FUNCTION_BLOCK "IMAC_STANDBY"
TITLE = STANDBY
//--------------------------------------------------------------------------------
//SIEMENS AG     I&S IP PEP SNPSP-Element: D-09300081-E-E5
//--------------------------------------------------------------------------------
//History
//=======
//  Date    Version  Description                     Author        CheckedReleased
//1997/06/09   0.6   Basic Edition                   Salge
//2004/11/25   1.0   Basic Edition converted to S7   Edelmann
//2004/12/02   1.1   Reset Timer in normal C/O       Edelmann
//--------------------------------------------------------------------------------
//PLC:   >= S7-300
//--------------------------------------------------------------------------------
//Specification:   Refer "TECHFUNK.DOC"
//--------------------------------------------------------------------------------
//Called FC : FC90 "DELAYTIMER"
//            SFC20 "BLKMOV"
//References: DB90.DBX3.1  (1 sec tact)
//--------------------------------------------------------------------------------
//at run time:
//--------------------------------------------------------------------------------
//
//--------------------------------------------------------------------------------
//Note:
//--------------------------------------------------------------------------------
// KNOW_HOW_PROTECT
AUTHOR : Sa_Edm
FAMILY : IMAC
NAME : STANDBY
VERSION : 1.0


VAR_INPUT
  OBJ : INT ;
  C_O : BOOL ;	//Changeover
  GSTA : BOOL ;	//Group start
  GSTO : BOOL ;	//Group stop
  FALT : BOOL ;	//Fault
  STAA : WORD ;	//Status motor A
  STAB : WORD ;	//Status motor B
  PCONF : STRUCT
   LastRecord : INT  := 100;
   Pointer1stRecord : STRUCT
    S7ID : BYTE  := B#16#10;	//ANY pointer: ID S7
    Typ : BYTE  := B#16#2;	//ANY pointer: data typ =02 BYTE =04 WORD =05 INT =06 DWORD =07 DINT =08 REAL
    RepeatFactor : INT  := 74;	//ANY pointer: repeat factor
    DBNo : INT  := 84;	//ANY pointer: DB number, zero if no DB
    MemoryArea : BYTE  := B#16#84;	//ANY pointer: Memory area =81 IN =82 OUT =83 M =84 DB =85 DI =86 L
    DWHigh : BYTE ;	//ANY pointer: DW highest byte
    DWX : INT ;	//ANY pointer: DW low / bit (address = byte *8 + bit)
   END_STRUCT ;
  END_STRUCT ;
END_VAR
VAR_OUTPUT
  ENAB : WORD ;
  ACOA : WORD ;	//ACOM motor A
  ACOB : WORD ;	//ACOM motor A
  OSSTAT : WORD ;	//Status for OS
  OSALARM : WORD ;	//Alarms for OS
END_VAR
VAR_IN_OUT
  OSCOM : WORD ;
END_VAR
VAR
  STANDBY : STRUCT
   System : WORD ;
   CmdOS : WORD ;
   MirrorCmdOS : WORD ;
   Test : WORD ;
   AlarmOS : WORD ;
   StatusOS : WORD ;
   SysStatusOS : WORD ;
   Status1 : WORD ;
   Status2 : WORD ;
   Status3 : BYTE ;
   InputEdges : BYTE ;
   AutoEdges : WORD ;
   DataTimeCODelay : STRUCT
    StartTime : DINT ;
    StartEdge : BOOL ;
   END_STRUCT ;
   DataTimeStartingA : STRUCT
    StartTime : DINT ;
    StartEdge : BOOL ;
   END_STRUCT ;
   DataTimeStartingB : STRUCT
    StartTime : DINT ;
    StartEdge : BOOL ;
   END_STRUCT ;
   DataTimeFaultA : STRUCT
    StartTime : DINT ;
    StartEdge : BOOL ;
   END_STRUCT ;
   DataTimeFaultB : STRUCT
    StartTime : DINT ;
    StartEdge : BOOL ;
   END_STRUCT ;
   PCONF : STRUCT
    Modeswitches : STRUCT
     M0_Spare : BOOL ;	// Spare
     M1_Spare : BOOL ;	// Spare
     M2_Spare : BOOL ;	// Spare
     M3_Spare : BOOL ;	// Spare
     M4_Spare : BOOL ;	// Spare
     M5_Spare : BOOL ;	// Spare
     M6_Spare : BOOL ;	// Spare
     M7_Spare : BOOL ;	// Spare
     M8_Spare : BOOL ;	// Spare
     M9_Spare : BOOL ;	// Spare
     M10_Spare : BOOL ;	// Spare
     M11_Spare : BOOL ;	// Spare
     M12_Spare : BOOL ;	// Spare
     M13_Spare : BOOL ;	// Spare
     M14_Spare : BOOL ;	// Spare
     M15_Test : BOOL ;	// Testbit (1)
    END_STRUCT ;
    DlyTCODelay : TIME ;	// Setpoint Action Fault delay
    DlyTStartingA : TIME ;	// Setpoint Waiting Delay Slow->Fast
    DlyTStartingB : TIME ;	// Setpoint Waiting Delay Fast->Slow
    DlyTFaultA : TIME ;	// Setpoint feedback fault delay
    DlyTFaultB : TIME ;	// Setpoint change direction
   END_STRUCT ;
  END_STRUCT ;
  siFailRR : INT ;	//Falure blockmove readrecord
  siFailWR : INT ;	//Failure blokmove write record
END_VAR
VAR_TEMP
  M200_0 : BOOL ;
  M200_1 : BOOL ;
  M200_2 : BOOL ;
  M200_3 : BOOL ;
  M200_4 : BOOL ;
  M200_5 : BOOL ;
  M200_6 : BOOL ;
  M200_7 : BOOL ;
  tbCmdCO : BOOL ;
  tbCmdStop : BOOL ;
  M201_2 : BOOL ;
  M201_3 : BOOL ;
  M201_4 : BOOL ;
  M201_5 : BOOL ;
  M201_6 : BOOL ;
  M201_7 : BOOL ;
  M202_0 : BOOL ;
  M202_1 : BOOL ;
  M202_2 : BOOL ;
  M202_3 : BOOL ;
  M202_4 : BOOL ;
  M202_5 : BOOL ;
  M202_6 : BOOL ;
  M202_7 : BOOL ;
  M203_0 : BOOL ;
  M203_1 : BOOL ;
  M203_2 : BOOL ;
  M203_3 : BOOL ;
  M203_4 : BOOL ;
  M203_5 : BOOL ;
  M203_6 : BOOL ;
  M203_7 : BOOL ;
  M204_0 : BOOL ;
  M204_1 : BOOL ;
  M204_2 : BOOL ;
  M204_3 : BOOL ;
  M204_4 : BOOL ;
  M204_5 : BOOL ;
  M204_6 : BOOL ;
  M204_7 : BOOL ;
  M205_0 : BOOL ;
  M205_1 : BOOL ;
  M205_2 : BOOL ;
  M205_3 : BOOL ;
  M205_4 : BOOL ;
  M205_5 : BOOL ;
  M205_6 : BOOL ;
  M205_7 : BOOL ;
  tbChangeover : BOOL ;
  tbGroupstart : BOOL ;
  tbGroupStop : BOOL ;
  tbExternalFault : BOOL ;
  M206_4 : BOOL ;
  M206_5 : BOOL ;
  M206_6 : BOOL ;
  M206_7 : BOOL ;
  M207_0 : BOOL ;
  M207_1 : BOOL ;
  M207_2 : BOOL ;
  M207_3 : BOOL ;
  M207_4 : BOOL ;
  M207_5 : BOOL ;
  M207_6 : BOOL ;
  M207_7 : BOOL ;
  M208_0 : BOOL ;
  M208_1 : BOOL ;
  M208_2 : BOOL ;
  M208_3 : BOOL ;
  M208_4 : BOOL ;
  M208_5 : BOOL ;
  M208_6 : BOOL ;
  M208_7 : BOOL ;
  M209_0 : BOOL ;
  M209_1 : BOOL ;
  M209_2 : BOOL ;
  M209_3 : BOOL ;
  M209_4 : BOOL ;
  M209_5 : BOOL ;
  M209_6 : BOOL ;
  M209_7 : BOOL ;
  M210_0 : BOOL ;
  M210_1 : BOOL ;
  M210_2 : BOOL ;
  M210_3 : BOOL ;
  M210_4 : BOOL ;
  M210_5 : BOOL ;
  M210_6 : BOOL ;
  M210_7 : BOOL ;
  M211_0 : BOOL ;
  M211_1 : BOOL ;
  M211_2 : BOOL ;
  M211_3 : BOOL ;
  M211_4 : BOOL ;
  M211_5 : BOOL ;
  M211_6 : BOOL ;
  M211_7 : BOOL ;
  M212_0 : BOOL ;
  M212_1 : BOOL ;
  M212_2 : BOOL ;
  M212_3 : BOOL ;
  M212_4 : BOOL ;
  M212_5 : BOOL ;
  M212_6 : BOOL ;
  M212_7 : BOOL ;
  M213_0 : BOOL ;
  M213_1 : BOOL ;
  M213_2 : BOOL ;
  M213_3 : BOOL ;
  M213_4 : BOOL ;
  M213_5 : BOOL ;
  M213_6 : BOOL ;
  M213_7 : BOOL ;
  tbMotAStarttimeOver : BOOL ;
  tbMotBStarttimeOver : BOOL ;
  tbCmdBlackoutStartA : BOOL ;
  tbCmdBlackoutStartB : BOOL ;
  tbCmdDelayStopA : BOOL ;
  tbCmdDelayStopB : BOOL ;
  M214_6 : BOOL ;
  M214_7 : BOOL ;
  tbOutStartA : BOOL ;
  tbOutStartB : BOOL ;
  tbOutStopA : BOOL ;
  tbOutStopB : BOOL ;
  tbLastMotWasA : BOOL ;
  tbLastMotWasB : BOOL ;
  tbChangeOverDelayAct : BOOL ;
  M215_7 : BOOL ;
  M216_0 : BOOL ;
  M216_1 : BOOL ;
  M216_2 : BOOL ;
  M216_3 : BOOL ;
  M216_4 : BOOL ;
  M216_5 : BOOL ;
  M216_6 : BOOL ;
  M216_7 : BOOL ;
  tbMotAAutoFailure : BOOL ;
  tbMotBAutoFailure : BOOL ;
  tbMotAFaulttimeActive : BOOL ;
  tbMotBFaulttimeActive : BOOL ;
  M217_4 : BOOL ;
  M217_5 : BOOL ;
  M217_6 : BOOL ;
  M217_7 : BOOL ;
  tbCmdCOPulse : BOOL ;
  tbCmdGSTAPulse : BOOL ;
  tbCmdGSTOPulse : BOOL ;
  M218_3 : BOOL ;
  M218_4 : BOOL ;
  M218_5 : BOOL ;
  M218_6 : BOOL ;
  M218_7 : BOOL ;
  M219_0 : BOOL ;
  M219_1 : BOOL ;
  M219_2 : BOOL ;
  M219_3 : BOOL ;
  M219_4 : BOOL ;
  M219_5 : BOOL ;
  M219_6 : BOOL ;
  M219_7 : BOOL ;
  M220_0 : BOOL ;
  M220_1 : BOOL ;
  M220_2 : BOOL ;
  M220_3 : BOOL ;
  M220_4 : BOOL ;
  M220_5 : BOOL ;
  M220_6 : BOOL ;
  M220_7 : BOOL ;
  M221_0 : BOOL ;
  M221_1 : BOOL ;
  M221_2 : BOOL ;
  M221_3 : BOOL ;
  M221_4 : BOOL ;
  M221_5 : BOOL ;
  M221_6 : BOOL ;
  M221_7 : BOOL ;
  tbAutoBlackoutstart : BOOL ;
  tbMotAStbyCtrl : BOOL ;
  M222_2 : BOOL ;
  M222_3 : BOOL ;
  M222_4 : BOOL ;
  M222_5 : BOOL ;
  M222_6 : BOOL ;
  tbMotAFetchData : BOOL ;
  tbMotAAutoStart : BOOL ;
  tbMotAAutoStop : BOOL ;
  tbMotAAutoFailure_1 : BOOL ;
  M223_3 : BOOL ;
  M223_4 : BOOL ;
  M223_5 : BOOL ;
  M223_6 : BOOL ;
  M223_7 : BOOL ;
  tbMotBlackoutstart : BOOL ;
  tbMotBStbyCtrl : BOOL ;
  M224_2 : BOOL ;
  M224_3 : BOOL ;
  M224_4 : BOOL ;
  M224_5 : BOOL ;
  M224_6 : BOOL ;
  tbMotBFetchData : BOOL ;
  tbMotBAutoStart : BOOL ;
  tbMotBAutoStop : BOOL ;
  tbMOtBAutoFailure_1 : BOOL ;
  M225_3 : BOOL ;
  M225_4 : BOOL ;
  M225_5 : BOOL ;
  M225_6 : BOOL ;
  M225_7 : BOOL ;
  M226_0 : BOOL ;
  M226_1 : BOOL ;
  M226_2 : BOOL ;
  M226_3 : BOOL ;
  M226_4 : BOOL ;
  M226_5 : BOOL ;
  M226_6 : BOOL ;
  M226_7 : BOOL ;
  tbMotARunning : BOOL ;
  tbMotALocal : BOOL ;
  tbMotAManual : BOOL ;
  tbMotAAuto : BOOL ;
  tbMotAFailure : BOOL ;
  tbMotABlackout : BOOL ;
  tbMotAFeedback : BOOL ;
  tbMotARestarting : BOOL ;
  M228_0 : BOOL ;
  M228_1 : BOOL ;
  M228_2 : BOOL ;
  M228_3 : BOOL ;
  M228_4 : BOOL ;
  M228_5 : BOOL ;
  M228_6 : BOOL ;
  M228_7 : BOOL ;
  tbMotBRunning : BOOL ;
  tbMotBLocal : BOOL ;
  tbMotBManual : BOOL ;
  tbMotBAuto : BOOL ;
  tbMotBFailure : BOOL ;
  tbMotBBlackout : BOOL ;
  tbMotBFeedback : BOOL ;
  tbMotBRestarting : BOOL ;
  P_currentRecord : ANY ;	//ANY pointer of the current record
END_VAR
BEGIN
NETWORK
TITLE =Calculation of current ANY pointer for reading /writing record
// ANY-pointer of current record
      L     #PCONF.Pointer1stRecord.S7ID;
      T     LB    30;
      L     #PCONF.Pointer1stRecord.Typ;
      T     LB    31;
      L     #PCONF.Pointer1stRecord.RepeatFactor;
      T     LW    32;
      L     #PCONF.Pointer1stRecord.DBNo;
      T     LW    34;
      L     #PCONF.Pointer1stRecord.MemoryArea;
      T     LB    36;
      L     #PCONF.Pointer1stRecord.DWHigh;
      T     LB    37;
      L     #PCONF.Pointer1stRecord.DWX;
      T     LW    38;

      L     #OBJ; //Check whether Obj within the range
      L     #PCONF.LastRecord;
      >I    ;
      SPB   cRcd;
      L     #OBJ;
      L     1;
      <I    ;
      SPB   cRcd;
      L     #OBJ;
cRcd: +     -1;
      L     #PCONF.Pointer1stRecord.RepeatFactor;
      *I    ;
      SLD   3; //DBW + DBX address of the current record
      L     LD    36;
      OD    ;
      T     LD    36; //DBWX part of ANY pointer "P_currentRecord"

NETWORK
TITLE =Read  record

      CALL "BLKMOV" (
           SRCBLK                   := #P_currentRecord,
           RET_VAL                  := #siFailRR,
           DSTBLK                   := #STANDBY);

NETWORK
TITLE =Read OS command

      L     #OSCOM; // Commands from OS
      T     LW     0;
      L     #STANDBY.Status1; // Status stored
      T     LW    14;
      L     #STANDBY.Status2; // Status stored
      T     LW    16;

      L     0; //Reset scratch  flags
      T     LW     6;
      T     LW    22;
      T     LW    24;
      T     LW    50;
      T     LW    52;
      T     LW    54;
NETWORK
TITLE =Formaloperanden Inputs

      U     #C_O;
      =     #tbChangeover; // Changeover
      U     #GSTA;
      =     #tbGroupstart; // Extern Groupstart
      U     #GSTO;
      =     #tbGroupStop; // Extern Groupstop
      U     #FALT;
      =     #tbExternalFault; // Extern Fault

      L     #STAA; // Status motor A
      T     LW    26;
      L     #STAB; // Status motor B
      T     LW    28;

// ----Evaluate Pulsflags from Auto Commands----
      L     #STANDBY.AutoEdges; //Stored Auto Command last cycle
      INVI  ; //Singlecomplement
      L     LW     6; //Command From Automatic
      T     #STANDBY.AutoEdges;
      UW    ;
      T     LW    18; // Command  Pulseflags
NETWORK
TITLE =Last Running Motor
//Setze den Motor als zuletzt laufenden Motor welcher zuletzt lief oder wenn
//anderer Motor einen Blackout hat//
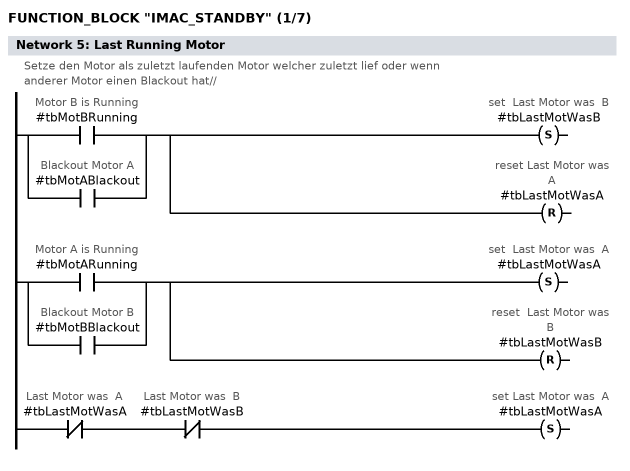
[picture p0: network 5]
      O     #tbMotBRunning; // Motor B is Running
      O     #tbMotABlackout; // Blackout Motor A
      S     #tbLastMotWasB; // set  Last Motor was  B
      R     #tbLastMotWasA; // reset Last Motor was  A

      O     #tbMotARunning; // Motor A is Running
      O     #tbMotBBlackout; // Blackout Motor B
      S     #tbLastMotWasA; // set  Last Motor was  A
      R     #tbLastMotWasB; // reset  Last Motor was  B

      UN    #tbLastMotWasA; // Last Motor was  A
      UN    #tbLastMotWasB; // Last Motor was  B
      S     #tbLastMotWasA; // set Last Motor was  A
NETWORK
TITLE =Commands
// ------- Start Last Running Motor----------
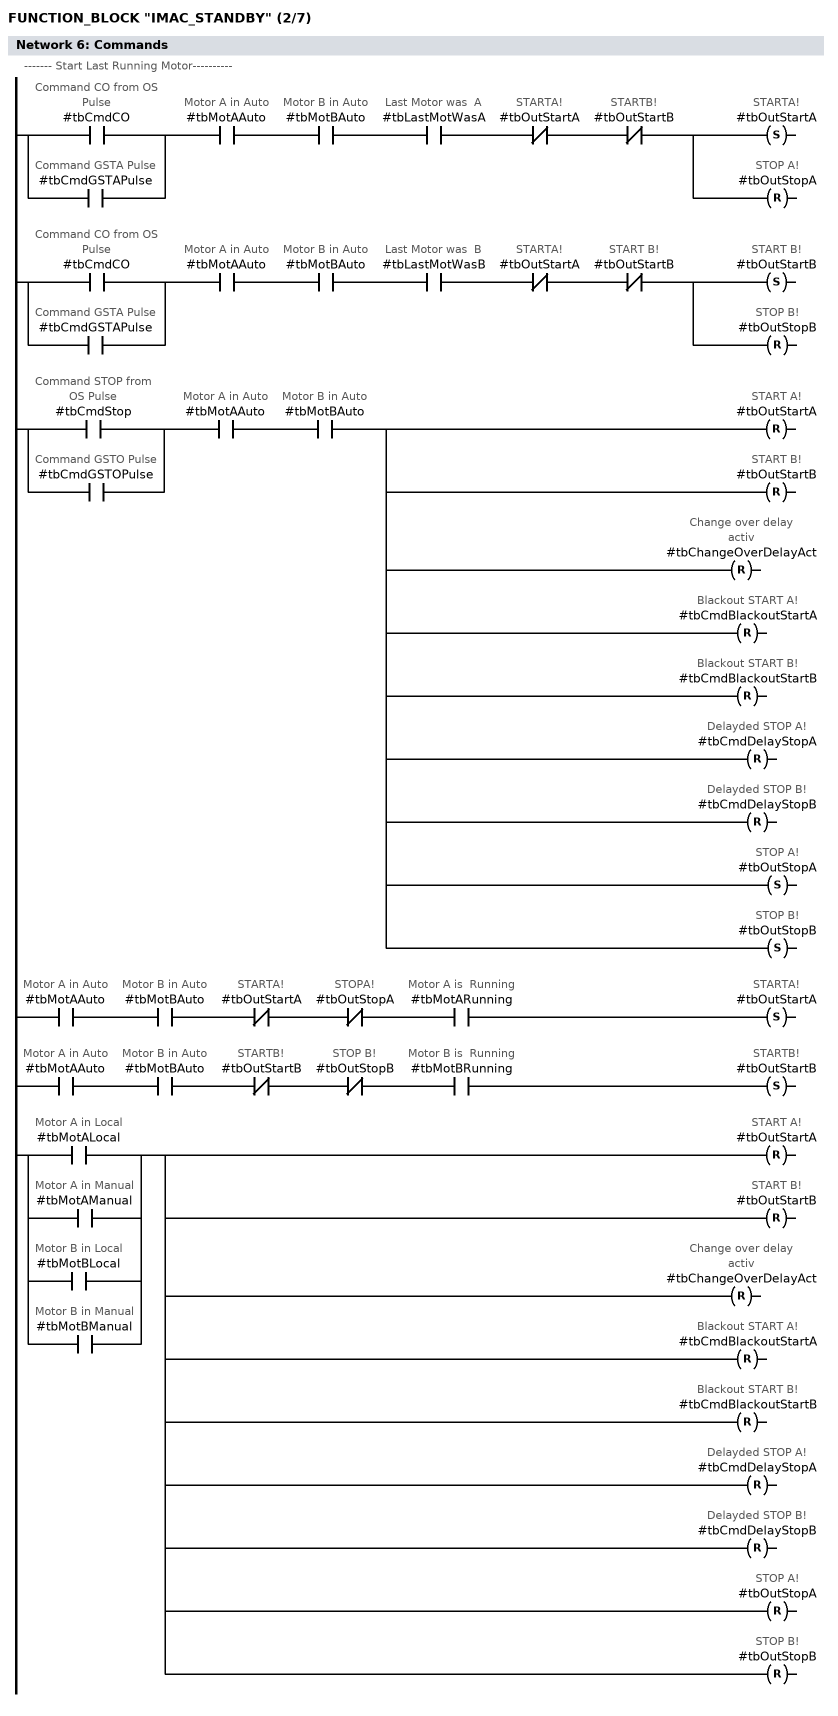
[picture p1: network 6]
      U(    ;
      O     #tbCmdCO; // Command CO from OS Pulse
      O     #tbCmdGSTAPulse; // Command GSTA Pulse
      )     ;
      U     #tbMotAAuto; // Motor A in Auto
      U     #tbMotBAuto; // Motor B in Auto
      U     #tbLastMotWasA; // Last Motor was  A
      UN    #tbOutStartA; // STARTA!
      UN    #tbOutStartB; // STARTB!
      S     #tbOutStartA; // STARTA!
      R     #tbOutStopA; // STOP A!

      U(    ;
      O     #tbCmdCO; // Command CO from OS Pulse
      O     #tbCmdGSTAPulse; // Command GSTA Pulse
      )     ;
      U     #tbMotAAuto; // Motor A in Auto
      U     #tbMotBAuto; // Motor B in Auto
      U     #tbLastMotWasB; // Last Motor was  B
      UN    #tbOutStartA; // STARTA!
      UN    #tbOutStartB; // START B!
      S     #tbOutStartB; // START B!
      R     #tbOutStopB; // STOP B!

// -------SET Stop Command----------
      U(    ;
      O     #tbCmdStop; // Command STOP from OS Pulse
      O     #tbCmdGSTOPulse; // Command GSTO Pulse
      )     ;
      U     #tbMotAAuto; // Motor A in Auto
      U     #tbMotBAuto; // Motor B in Auto
      R     #tbOutStartA; // START A!
      R     #tbOutStartB; // START B!
      R     #tbChangeOverDelayAct; // Change over delay activ
      R     #tbCmdBlackoutStartA; // Blackout START A!
      R     #tbCmdBlackoutStartB; // Blackout START B!
      R     #tbCmdDelayStopA; // Delayded STOP A!
      R     #tbCmdDelayStopB; // Delayded STOP B!
      S     #tbOutStopA; // STOP A!
      S     #tbOutStopB; // STOP B!

// ------- Manual to Auto change----------
      U     #tbMotAAuto; // Motor A in Auto
      U     #tbMotBAuto; // Motor B in Auto
      UN    #tbOutStartA; // STARTA!
      UN    #tbOutStopA; // STOPA!
      U     #tbMotARunning; // Motor A is  Running
      S     #tbOutStartA; // STARTA!

      U     #tbMotAAuto; // Motor A in Auto
      U     #tbMotBAuto; // Motor B in Auto
      UN    #tbOutStartB; // STARTB!
      UN    #tbOutStopB; // STOP B!
      U     #tbMotBRunning; // Motor B is  Running
      S     #tbOutStartB; // STARTB!

// ------- Reset all if Auto changed  to Manual or Local ----------
      O     #tbMotALocal; // Motor A in Local
      O     #tbMotAManual; // Motor A in Manual
      O     #tbMotBLocal; // Motor B in Local
      O     #tbMotBManual; // Motor B in Manual
      R     #tbOutStartA; // START A!
      R     #tbOutStartB; // START B!
      R     #tbChangeOverDelayAct; // Change over delay activ
      R     #tbCmdBlackoutStartA; // Blackout START A!
      R     #tbCmdBlackoutStartB; // Blackout START B!
      R     #tbCmdDelayStopA; // Delayded STOP A!
      R     #tbCmdDelayStopB; // Delayded STOP B!
      R     #tbOutStopA; // STOP A!
      R     #tbOutStopB; // STOP B!
NETWORK
TITLE =AutoFailure
// ---Starting Timer A-----
//--- Nach start des Motors A  wird eine Verzögertungszeit gestartet die die
//Weitergabe des externen Fehlereingengs  an A verzögert//
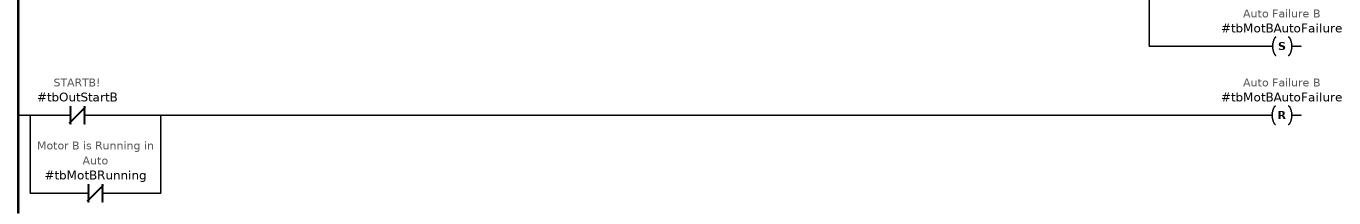
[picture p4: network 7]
      U     #tbOutStartA; // STARTA!
      U     #tbMotARunning; // Motor A is Running Iin Auto
      UN    #tbMotBFailure; // Motor B Failure
      UN    #tbMotAStarttimeOver; // Starting A time is over
      UN    #tbMotABlackout; // Motor A Blackout
      UN    #tbMotBBlackout; // Motor B Blackout
      =     L     50.1; // Starting A activ

//Starting A timer
      CALL "IMAC_DELAYTIMER" (
           XSTART                   := L     50.1,// Starting A timer activ
           XTIME                    := #STANDBY.PCONF.DlyTStartingA,
           YON                      := L     50.2,
           MEM                      := #STANDBY.DataTimeStartingA);

      U     L     50.2; // Time is over
      S     #tbMotAStarttimeOver; // Starting A time is over
      ON    #tbOutStartA; // STARTA!
      ON    #tbMotARunning; // Motor A is Running in Auto
      O     #tbMotABlackout; // Motor A Blackout
      O     #tbMotBBlackout; // Motor B Blackout
      R     #tbMotAStarttimeOver; // Starting A time is over

//--- Nach start des Motors B wird eine Verzögertungszeit gestartet die die Weitergabe des Externen Fehlereingengs  an B verzögert//
      U     #tbOutStartB; // STARTB!
      U     #tbMotBRunning; // Motor B is Running Iin Auto
      UN    #tbMotAFailure; // Motor A Failure
      UN    #tbMotBStarttimeOver; // Starting B time is over
      UN    #tbMotABlackout; // Motor A Blackout
      UN    #tbMotBBlackout; // Motor B Blackout
      =     L     50.3; // Starting B activ

//Starting B timer
      CALL "IMAC_DELAYTIMER" (
           XSTART                   := L     50.3,// Starting B timer activ
           XTIME                    := #STANDBY.PCONF.DlyTStartingB,
           YON                      := L     50.4,
           MEM                      := #STANDBY.DataTimeStartingB);

      U     L     50.4; // Time is over
      S     #tbMotBStarttimeOver; // Starting B time is over
      ON    #tbOutStartB; // STARTB!
      ON    #tbMotBRunning; // Motor B is Running in Auto
      O     #tbMotABlackout; // Motor A Blackout
      O     #tbMotBBlackout; // Motor B Blackout
      R     #tbMotBStarttimeOver; // Starting B time is over
//---External Fault Verzoegerung wenn Starting time A abgelaufen
      L     20;
      T     #STANDBY.DataTimeFaultA.StartTime;

      U     #tbMotAStarttimeOver; // Starting A time is over
      U     #tbExternalFault; // External Fault input
      =     #tbMotAFaulttimeActive; // Fault timer A activ

//Fault timer A
      CALL "IMAC_DELAYTIMER" (
           XSTART                   := #tbMotAFaulttimeActive,// Fault timer A activ
           XTIME                    := #STANDBY.PCONF.DlyTFaultA,
           YON                      := L     50.5,
           MEM                      := #STANDBY.DataTimeFaultA);

//----Change over von A nach B

      U     L     50.5; // External Fault time over pulse
      U     #tbMotAStarttimeOver; // Starting A time is over
      U     #tbMotAAuto; // Motor A in Auto
      U     #tbMotBAuto; // Motor B in Auto
      U     #tbOutStartA; // STARTA!
      U     #tbMotARunning; // Motor A is Running
      UN    #tbOutStartB; // STARTB!
      UN    #tbMotBRunning; // Motor B is Running
      UN    #tbMotBFailure; // Motor B Failure
      UN    #tbMotBBlackout; // Motor B Blackout
      S     #tbOutStartB; // STARTB!
      S     #tbChangeOverDelayAct; // Change over delay activ
      S     #tbCmdDelayStopA; // Delayded STOP A!
      R     #tbCmdDelayStopB; // Delayded STOP B!
      S     #tbMotAAutoFailure; // Auto Failure A
      ON    #tbOutStartA; // STARTA!
      ON    #tbMotARunning; // Motor A is Running in Auto
      R     #tbMotAAutoFailure; // Auto Failure A

//---External Fault Verzoegerung wenn Starting time  B abgelaufen
      L     20;
      T     #STANDBY.DataTimeFaultB.StartTime;

      U     #tbMotBStarttimeOver; // Starting B time is over
      U     #tbExternalFault; // External Fault input
      =     #tbMotBFaulttimeActive; // Fault timer B activ

//Fault timer B
      CALL "IMAC_DELAYTIMER" (
           XSTART                   := #tbMotBFaulttimeActive,// Fault timer B activ
           XTIME                    := #STANDBY.PCONF.DlyTFaultB,
           YON                      := L     50.6,
           MEM                      := #STANDBY.DataTimeFaultB);

//----Change from Motor B to Motor A-------
      U     L     50.6; // External Fault time over pulse
      U     #tbMotBStarttimeOver; // Starting B time is over
      U     #tbMotAAuto; // Motor A in Auto
      U     #tbMotBAuto; // Motor B in Auto
      U     #tbOutStartB; // STARTB!
      U     #tbMotBRunning; // Motor B is Running
      UN    #tbOutStartA; // STARTA!
      UN    #tbMotARunning; // Motor A is Running
      UN    #tbMotAFailure; // Motor A Failure
      UN    #tbMotABlackout; // Motor A Blackout
      S     #tbOutStartA; // STARTA!
      S     #tbChangeOverDelayAct; // Change over delay activ
      S     #tbCmdDelayStopB; // Delayded STOP B!
      R     #tbCmdDelayStopA; // Delayded STOP A!
      S     #tbMotBAutoFailure; // Auto Failure B
      ON    #tbOutStartB; // STARTB!
      ON    #tbMotBRunning; // Motor B is Running in Auto
      R     #tbMotBAutoFailure; // Auto Failure B
NETWORK
TITLE =Normal Change Over
//----Change from Motor A to Motor B-------
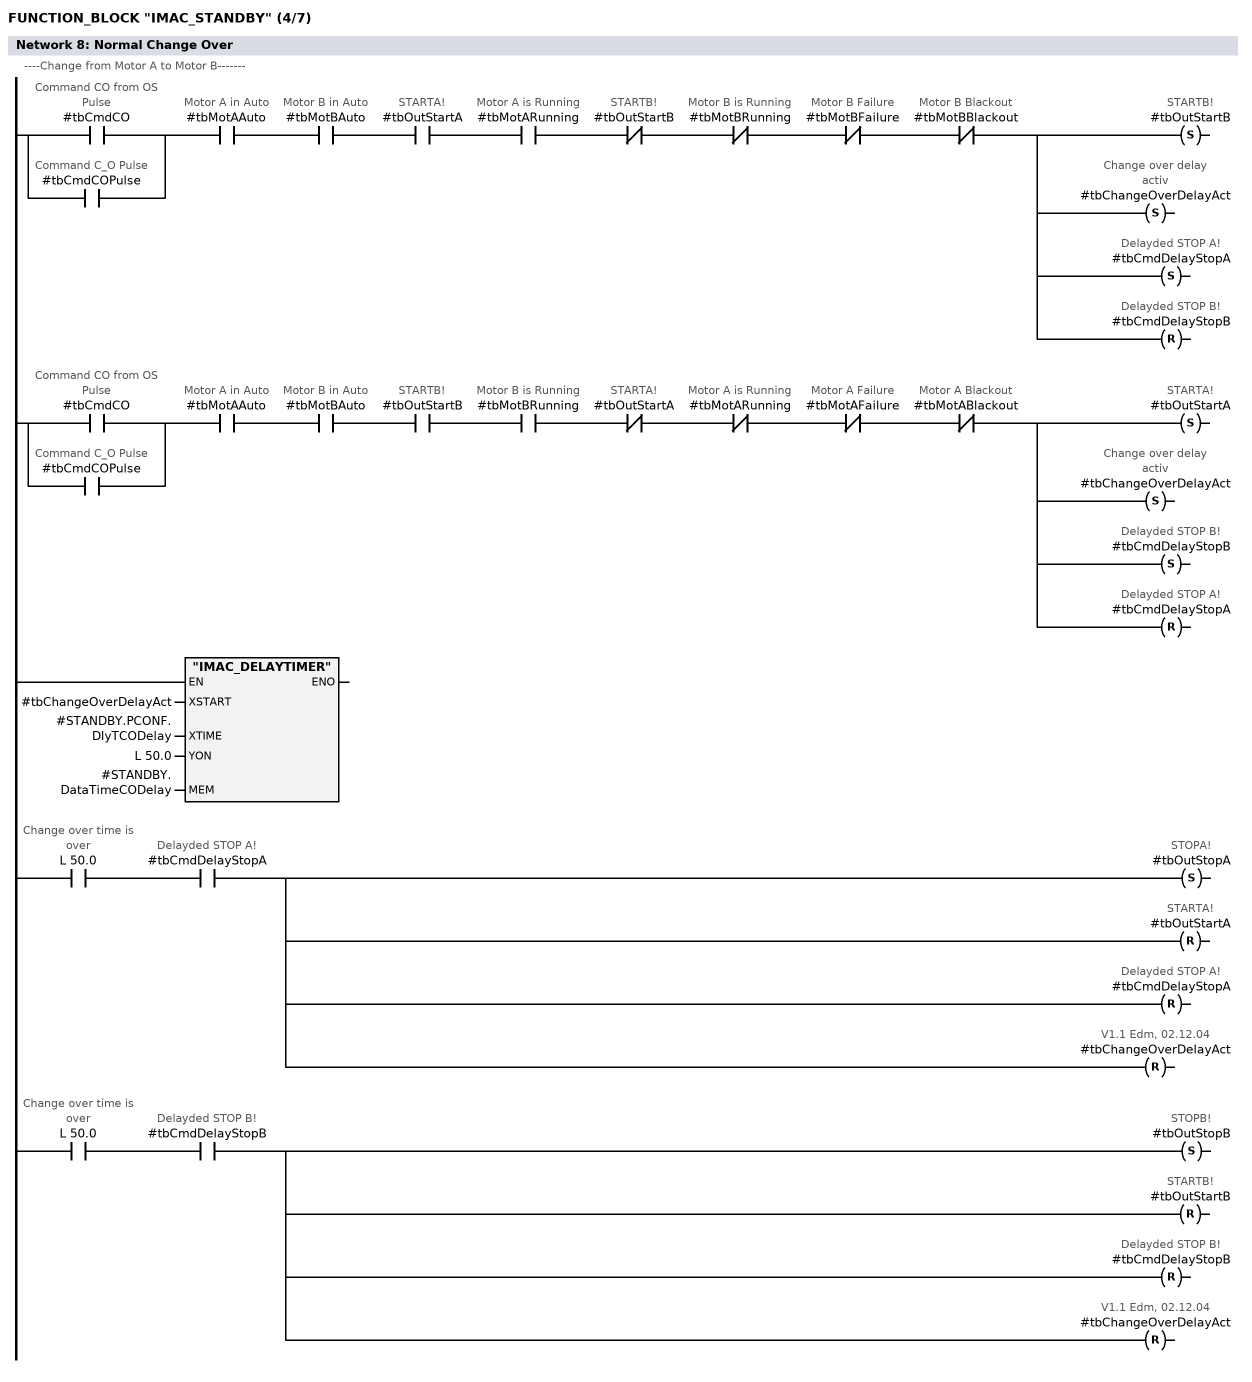
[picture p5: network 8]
      U(    ;
      O     #tbCmdCO; // Command CO from OS Pulse
      O     #tbCmdCOPulse; // Command C_O Pulse
      )     ;
      U     #tbMotAAuto; // Motor A in Auto
      U     #tbMotBAuto; // Motor B in Auto
      U     #tbOutStartA; // STARTA!
      U     #tbMotARunning; // Motor A is Running
      UN    #tbOutStartB; // STARTB!
      UN    #tbMotBRunning; // Motor B is Running
      UN    #tbMotBFailure; // Motor B Failure
      UN    #tbMotBBlackout; // Motor B Blackout
      S     #tbOutStartB; // STARTB!
      S     #tbChangeOverDelayAct; // Change over delay activ
      S     #tbCmdDelayStopA; // Delayded STOP A!
      R     #tbCmdDelayStopB; // Delayded STOP B!

//----Change from Motor B to Motor A-------
      U(    ;
      O     #tbCmdCO; // Command CO from OS Pulse
      O     #tbCmdCOPulse; // Command C_O Pulse
      )     ;
      U     #tbMotAAuto; // Motor A in Auto
      U     #tbMotBAuto; // Motor B in Auto
      U     #tbOutStartB; // STARTB!
      U     #tbMotBRunning; // Motor B is Running
      UN    #tbOutStartA; // STARTA!
      UN    #tbMotARunning; // Motor A is Running
      UN    #tbMotAFailure; // Motor A Failure
      UN    #tbMotABlackout; // Motor A Blackout
      S     #tbOutStartA; // STARTA!
      S     #tbChangeOverDelayAct; // Change over delay activ
      S     #tbCmdDelayStopB; // Delayded STOP B!
      R     #tbCmdDelayStopA; // Delayded STOP A!

//----Change over timer-------
//Change over time
      CALL "IMAC_DELAYTIMER" (
           XSTART                   := #tbChangeOverDelayAct,// Change over time activ
           XTIME                    := #STANDBY.PCONF.DlyTCODelay,
           YON                      := L     50.0,
           MEM                      := #STANDBY.DataTimeCODelay);

      U     L     50.0; //Change over time is over
      U     #tbCmdDelayStopA; // Delayded STOP A!
      S     #tbOutStopA; // STOPA!
      R     #tbOutStartA; // STARTA!
      R     #tbCmdDelayStopA; // Delayded STOP A!
      R     #tbChangeOverDelayAct; // V1.1 Edm, 02.12.04
      U     L     50.0; //Change over time is over
      U     #tbCmdDelayStopB; // Delayded STOP B!
      S     #tbOutStopB; // STOPB!
      R     #tbOutStartB; // STARTB!
      R     #tbCmdDelayStopB; // Delayded STOP B!
      R     #tbChangeOverDelayAct; // V1.1 Edm, 02.12.04
NETWORK
TITLE =Change Over IF Failure
//----Change from Motor A to Motor B-------
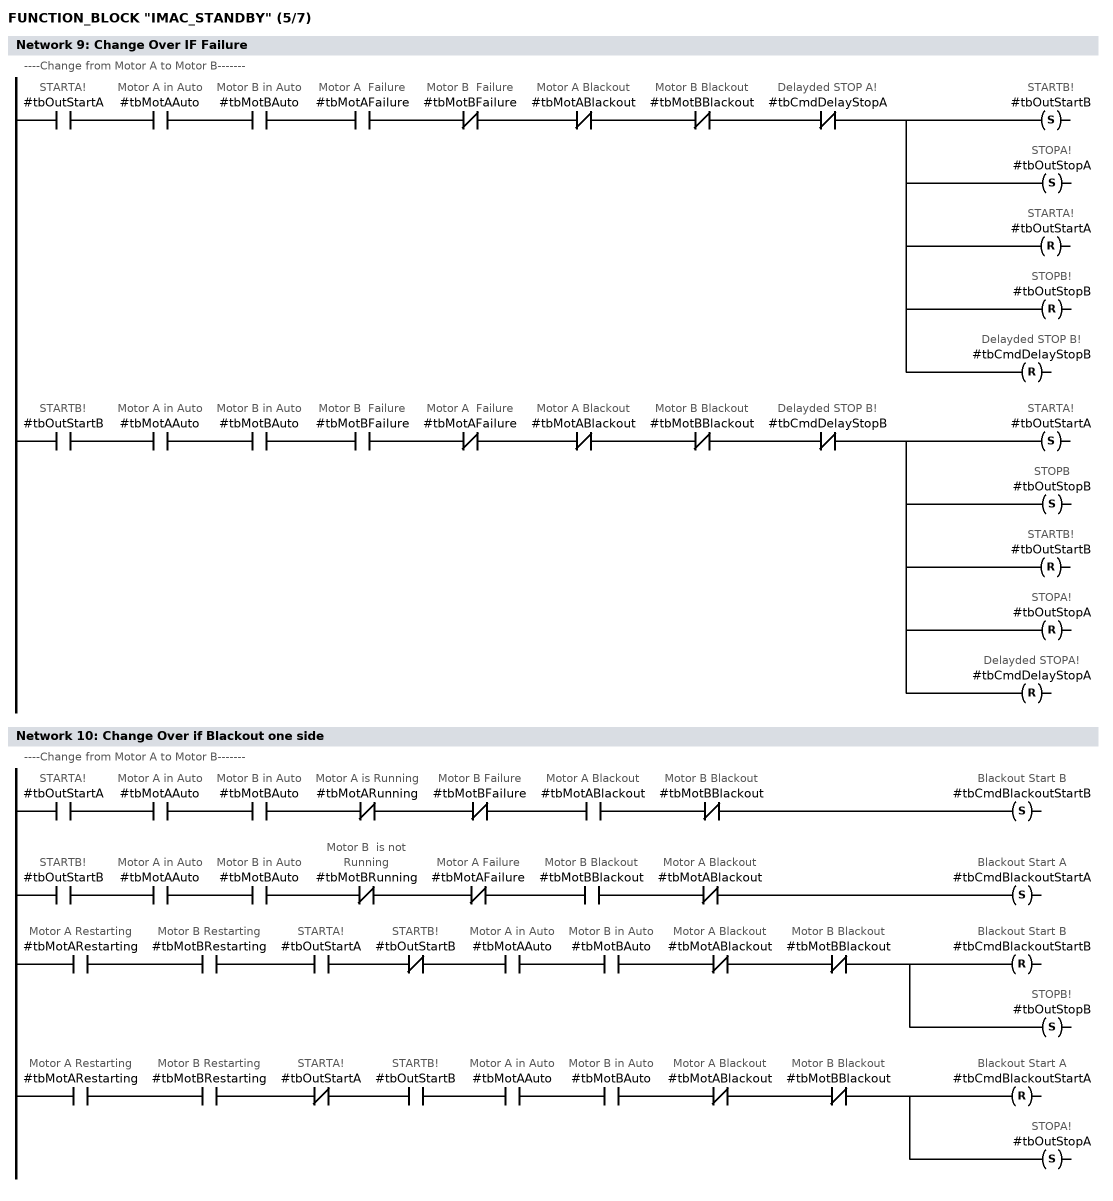
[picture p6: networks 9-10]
      U     #tbOutStartA; // STARTA!
      U     #tbMotAAuto; // Motor A in Auto
      U     #tbMotBAuto; // Motor B in Auto
      U     #tbMotAFailure; // Motor A  Failure
      UN    #tbMotBFailure; // Motor B  Failure
      UN    #tbMotABlackout; // Motor A Blackout
      UN    #tbMotBBlackout; // Motor B Blackout
      UN    #tbCmdDelayStopA; // Delayded STOP A!
      S     #tbOutStartB; // STARTB!
      S     #tbOutStopA; // STOPA!
      R     #tbOutStartA; // STARTA!
      R     #tbOutStopB; // STOPB!
      R     #tbCmdDelayStopB; // Delayded STOP B!

//----Change from Motor B to Motor A-------

      U     #tbOutStartB; // STARTB!
      U     #tbMotAAuto; // Motor A in Auto
      U     #tbMotBAuto; // Motor B in Auto
      U     #tbMotBFailure; // Motor B  Failure
      UN    #tbMotAFailure; // Motor A  Failure
      UN    #tbMotABlackout; // Motor A Blackout
      UN    #tbMotBBlackout; // Motor B Blackout
      UN    #tbCmdDelayStopB; // Delayded STOP B!
      S     #tbOutStartA; // STARTA!
      S     #tbOutStopB; // STOPB
      R     #tbOutStartB; // STARTB!
      R     #tbOutStopA; // STOPA!
      R     #tbCmdDelayStopA; // Delayded STOPA!
NETWORK
TITLE =Change Over if Blackout one side
//----Change from Motor A to Motor B-------
      U     #tbOutStartA; // STARTA!
      U     #tbMotAAuto; // Motor A in Auto
      U     #tbMotBAuto; // Motor B in Auto
      UN    #tbMotARunning; // Motor A is Running
      UN    #tbMotBFailure; // Motor B Failure
      U     #tbMotABlackout; // Motor A Blackout
      UN    #tbMotBBlackout; // Motor B Blackout
      S     #tbCmdBlackoutStartB; // Blackout Start B

//----Change from Motor B to Motor A-------
      U     #tbOutStartB; // STARTB!
      U     #tbMotAAuto; // Motor A in Auto
      U     #tbMotBAuto; // Motor B in Auto
      UN    #tbMotBRunning; // Motor B  is not Running
      UN    #tbMotAFailure; // Motor A Failure
      U     #tbMotBBlackout; // Motor B Blackout
      UN    #tbMotABlackout; // Motor A Blackout
      S     #tbCmdBlackoutStartA; // Blackout Start A
//---- Reset Blackoutstart und stoppe Restarting des Standby motors wenn beide Motoren Restarten

      U     #tbMotARestarting; // Motor A Restarting
      U     #tbMotBRestarting; // Motor B Restarting
      U     #tbOutStartA; // STARTA!
      UN    #tbOutStartB; // STARTB!
      U     #tbMotAAuto; // Motor A in Auto
      U     #tbMotBAuto; // Motor B in Auto
      UN    #tbMotABlackout; // Motor A Blackout
      UN    #tbMotBBlackout; // Motor B Blackout
      R     #tbCmdBlackoutStartB; // Blackout Start B
      S     #tbOutStopB; // STOPB!


      U     #tbMotARestarting; // Motor A Restarting
      U     #tbMotBRestarting; // Motor B Restarting
      UN    #tbOutStartA; // STARTA!
      U     #tbOutStartB; // STARTB!
      U     #tbMotAAuto; // Motor A in Auto
      U     #tbMotBAuto; // Motor B in Auto
      UN    #tbMotABlackout; // Motor A Blackout
      UN    #tbMotBBlackout; // Motor B Blackout
      R     #tbCmdBlackoutStartA; // Blackout Start A
      S     #tbOutStopA; // STOPA!
NETWORK
TITLE =Reset Control
//---- One is running -------
//Wenn beide Motoren angewahlt sind aber einer bereits läuft  stoppe Anwahl des
//anderen Motors außer wenn Change over Zeit läuft
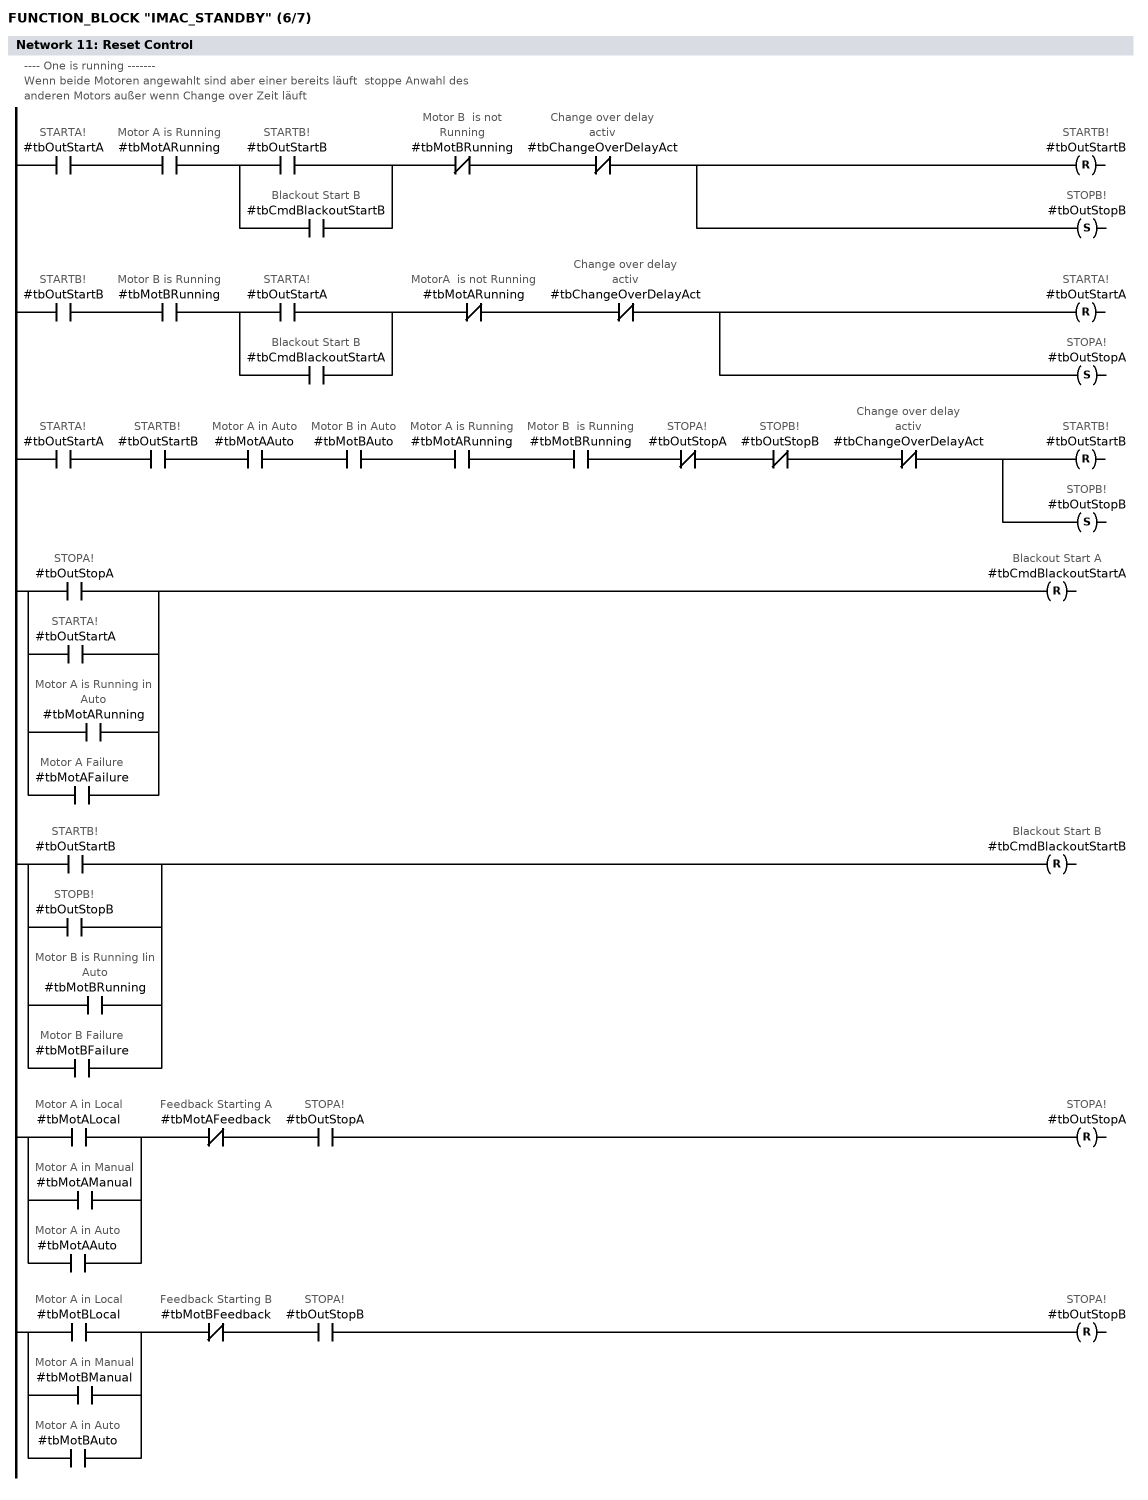
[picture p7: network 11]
      U     #tbOutStartA; // STARTA!
      U     #tbMotARunning; // Motor A is Running
      U(    ;
      O     #tbOutStartB; // STARTB!
      O     #tbCmdBlackoutStartB; // Blackout Start B
      )     ;
      UN    #tbMotBRunning; // Motor B  is not Running
      UN    #tbChangeOverDelayAct; // Change over delay activ
      R     #tbOutStartB; // STARTB!
      S     #tbOutStopB; // STOPB!
      U     #tbOutStartB; // STARTB!
      U     #tbMotBRunning; // Motor B is Running
      U(    ;
      O     #tbOutStartA; // STARTA!
      O     #tbCmdBlackoutStartA; // Blackout Start B
      )     ;
      UN    #tbMotARunning; // MotorA  is not Running
      UN    #tbChangeOverDelayAct; // Change over delay activ
      R     #tbOutStartA; // STARTA!
      S     #tbOutStopA; // STOPA!

//---- Both Are running -------
// Wenn Beide Motoren laufen und kein Motor abgeschaltet wird und auch kein Change over erfogt schalte MotorB ab//
      U     #tbOutStartA; // STARTA!
      U     #tbOutStartB; // STARTB!
      U     #tbMotAAuto; // Motor A in Auto
      U     #tbMotBAuto; // Motor B in Auto
      U     #tbMotARunning; // Motor A is Running
      U     #tbMotBRunning; // Motor B  is Running
      UN    #tbOutStopA; // STOPA!
      UN    #tbOutStopB; // STOPB!
      UN    #tbChangeOverDelayAct; // Change over delay activ
      R     #tbOutStartB; // STARTB!
      S     #tbOutStopB; // STOPB!

//---- Reset Blackoutstart -------
// Rücksete den verzögerten Startbefehl zum Motor wenn der Motor stoppen soll oderer laüft bereits oder er wird gestartet//
      O     #tbOutStopA; // STOPA!
      O     #tbOutStartA; // STARTA!
      O     #tbMotARunning; // Motor A is Running in Auto
      O     #tbMotAFailure; // Motor A Failure
      R     #tbCmdBlackoutStartA; // Blackout Start A


      O     #tbOutStartB; // STARTB!
      O     #tbOutStopB; // STOPB!
      O     #tbMotBRunning; // Motor B is Running Iin Auto
      O     #tbMotBFailure; // Motor B Failure
      R     #tbCmdBlackoutStartB; // Blackout Start B

//---- Reset STOP -------
// Rücksetze den Stop Befehl zum Motor wenn sicher keine Startoption im Motorbaustein ansteht und er nicht Laüft//
      O     #tbMotALocal; // Motor A in Local
      O     #tbMotAManual; // Motor A in Manual
      O     #tbMotAAuto; // Motor A in Auto
      UN    #tbMotAFeedback; //Feedback Starting A
      U     #tbOutStopA; // STOPA!
      R     #tbOutStopA; // STOPA!

      O     #tbMotBLocal; // Motor A in Local
      O     #tbMotBManual; // Motor A in Manual
      O     #tbMotBAuto; // Motor A in Auto
      UN    #tbMotBFeedback; //Feedback Starting B
      U     #tbOutStopB; // STOPA!
      R     #tbOutStopB; // STOPA!
NETWORK
TITLE =Automatic Outputs
//---- Commands to  MOTOR A -------
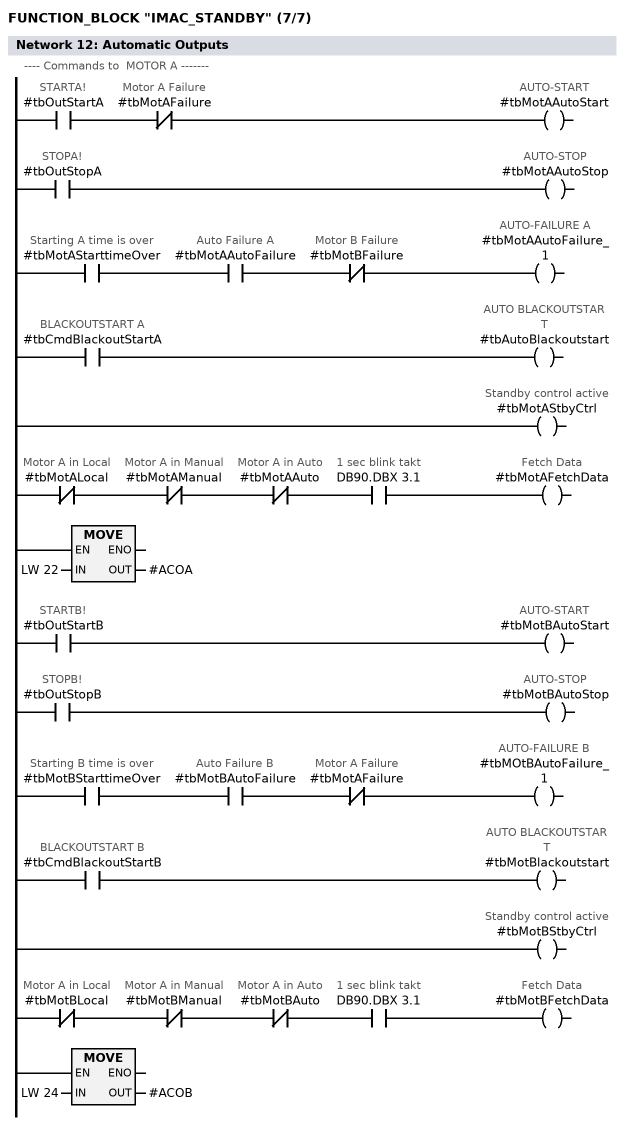
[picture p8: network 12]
      U     #tbOutStartA; // STARTA!
      UN    #tbMotAFailure; // Motor A Failure
      =     #tbMotAAutoStart; // AUTO-START
      U     #tbOutStopA; // STOPA!
      =     #tbMotAAutoStop; // AUTO-STOP
      U     #tbMotAStarttimeOver; // Starting A time is over
      U     #tbMotAAutoFailure; // Auto Failure A
      UN    #tbMotBFailure; // Motor B Failure
      =     #tbMotAAutoFailure_1; // AUTO-FAILURE A
      U     #tbCmdBlackoutStartA; // BLACKOUTSTART A
      =     #tbAutoBlackoutstart; // AUTO BLACKOUTSTART
      SET   ;
      =     #tbMotAStbyCtrl; //Standby control active
      UN    #tbMotALocal; // Motor A in Local
      UN    #tbMotAManual; // Motor A in Manual
      UN    #tbMotAAuto; // Motor A in Auto
      U     DB90.DBX    3.1; // 1 sec blink takt
      =     #tbMotAFetchData; // Fetch Data

      L     LW    22;
      T     #ACOA; //ACOM A

//---- Commands  to  MOTOR B -------

      U     #tbOutStartB; // STARTB!
      =     #tbMotBAutoStart; // AUTO-START
      U     #tbOutStopB; // STOPB!
      =     #tbMotBAutoStop; // AUTO-STOP
      U     #tbMotBStarttimeOver; // Starting B time is over
      U     #tbMotBAutoFailure; // Auto Failure B
      UN    #tbMotAFailure; // Motor A Failure
      =     #tbMOtBAutoFailure_1; // AUTO-FAILURE B
      U     #tbCmdBlackoutStartB; // BLACKOUTSTART B
      =     #tbMotBlackoutstart; // AUTO BLACKOUTSTART
      SET   ;
      =     #tbMotBStbyCtrl; //Standby control active
      UN    #tbMotBLocal; // Motor A in Local
      UN    #tbMotBManual; // Motor A in Manual
      UN    #tbMotBAuto; // Motor A in Auto
      U     DB90.DBX    3.1; // 1 sec blink takt
      =     #tbMotBFetchData; // Fetch Data

      L     LW    24;
      T     #ACOB; // ACOM B
NETWORK
TITLE =Combinate States
//----Alarms----
      U     #tbMotAStarttimeOver; // Starting A time is over
      U     #tbExternalFault; // External Fault input
      U     #tbMotBStarttimeOver; // Starting A time is over
      U     #tbExternalFault; // External Fault input
      L     2; //Fault Standby Alarm
      SPB   COD1;
      L     1; // Normal
COD1: T     LW    10; //States to OS

//----Status----
      ON    #tbMotAAuto; // Motor A in Auto
      ON    #tbMotBAuto; // Motor B in Auto
      L     1; // Stopped
      SPB   COD2;

      U     #tbMotAAuto; // Motor A in Auto
      U     #tbMotBAuto; // Motor B in Auto
      U     #tbOutStartB; // STARTB!
      U     #tbMotBRunning; // Motor B  is  Running
      UN    #tbOutStartA; // STARTA!
      UN    #tbMotARunning; // Motor A is Running
      UN    #tbMotAFailure; // Motor A Failure
      UN    #tbMotABlackout; // Motor A Blackout
      L     2; // Standby Motor A
      SPB   COD2;


      U     #tbMotAAuto; // Motor A in Auto
      U     #tbMotBAuto; // Motor B in Auto
      U     #tbOutStartA; // STARTA!
      U     #tbMotARunning; // Motor A is Running
      UN    #tbOutStartB; // STARTB!
      UN    #tbMotBRunning; // Motor B is Running
      UN    #tbMotBFailure; // Motor B Failure
      UN    #tbMotBBlackout; // Motor B Blackout
      L     3; // Standby Motor B
      SPB   COD2;
      L     0; //Undefined
COD2: T     LW    12; //States to OS
NETWORK
TITLE = Store States in Record

      L     0; // Reset Commands OS
      T     #STANDBY.CmdOS;
      T     #OSCOM; // Write Reset Back to I/O interface  added: 20060619 /Ho
      L     LW    10;
      T     #STANDBY.AlarmOS; // Alarms to OS
      T     #OSALARM;
      L     LW    12;
      T     #STANDBY.StatusOS; // States to OS
      T     #OSSTAT;
      L     LW    14;
      T     #STANDBY.Status1; // Status stored
      L     LW    16;
      T     #STANDBY.Status2; // Status stored
NETWORK
TITLE =Write record

      CALL "BLKMOV" (
           SRCBLK                   := #STANDBY,
           RET_VAL                  := #siFailWR,
           DSTBLK                   := #P_currentRecord);

END_FUNCTION_BLOCK

